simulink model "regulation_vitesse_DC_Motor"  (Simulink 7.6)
settings: Solver=ode23tb  StartTime=0.0  StopTime=0.4  RelTol=1e-3
PreLoadFcn:
  | close all
  | clc
  | clear all
PostLoadFcn:
  | Ki=1e-4;
  | Kd=1e-4;
  | Kp=5;
StopFcn:
  | close all, clc
  | load reg_vit.mat
  | plot(x(1,:),x(2,:), x(1,:),x(3,:))
  | grid
  | title('Consigne et sortie vitesse DC Motor')
  | xlabel('temps')
  | axis([0 0.4 0 1200])
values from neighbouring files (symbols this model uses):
  f = 1e-8    (= 1e-08)    [parametres.m]    (also in impedance_quartz.m = [1.59:0.0005:1.596]*1e6)
  R = 4    [parametres.m]    (also in Prog_callbacks.m = 1000; oscillateur_dephasage.m = 1000; Calcul_Ampl_phase_A.m = 1; circuit_RLC_parallele_.m)
undefined symbols (not defined in the file or in its folder): sigbuilder_block
libraries: fl_lib x19, nesl_utility x6

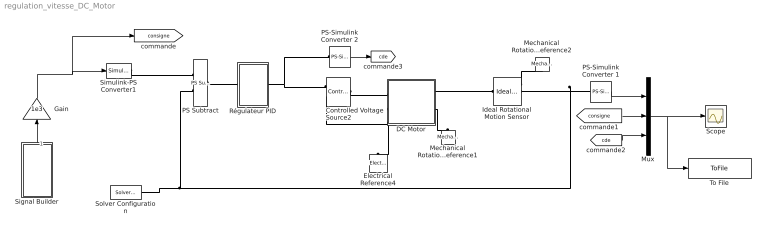
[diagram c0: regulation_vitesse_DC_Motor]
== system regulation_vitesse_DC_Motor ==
  Controlled Voltage Source2 : fl_lib/Electrical/Electrical Sources/Controlled Voltage Source  DialogController=NetworkEngine.DynNeDlgSource  SystemSampleTime=-1  i_Log=off  v_Log=off  LocalVarNames=|current|voltage|power  LocalVarDescs=|Current (A)|Voltage (V)|Power (W)  LocalVarLogging=[0 0 0]
  DC Motor : Subsystem  LoadFcn=|
      | R=4; % Résistance d'induit             
      | L=1e-5; % Inductance d'induit          
      | K=0.0005; % paramètre électromagnétique
      |                                        
      | J=1; %inertie (g*cm^2)                 
      | Cr=0.02e-3; % frottements              
      | f=1e-8; % amortissement
  Electrical Reference4 : fl_lib/Electrical/Electrical Elements/Electrical Reference  DialogController=NetworkEngine.DynNeDlgSource  SystemSampleTime=-1  i_Log=off  LocalVarNames=|i  LocalVarDescs=|i  LocalVarLogging=[]
  Gain : Gain  Gain=1e3
  Ideal Rotational Motion Sensor : fl_lib/Mechanical/Mechanical Sensors/Ideal Rotational Motion Sensor  DialogController=NetworkEngine.DynNeDlgSource  SystemSampleTime=-1  offset=0 rad  w_Log=off  t_Log=off  phi_Log=off  LocalVarNames=|w|t|phi  LocalVarDescs=|w|t|phi  LocalVarLogging=[0 0 0]
  Mechanical Rotational Reference1 : fl_lib/Mechanical/Rotational Elements/Mechanical Rotational Reference  DialogController=NetworkEngine.DynNeDlgSource  SystemSampleTime=-1  t_Log=off  LocalVarNames=|t  LocalVarDescs=|t  LocalVarLogging=[]
  Mechanical Rotational Reference2 : fl_lib/Mechanical/Rotational Elements/Mechanical Rotational Reference  DialogController=NetworkEngine.DynNeDlgSource  SystemSampleTime=-1  t_Log=off  LocalVarNames=|t  LocalVarDescs=|t  LocalVarLogging=[]
  Mux : Mux  Inputs=3
  PS Subtract : fl_lib/Physical Signals/Functions/PS Subtract  DialogController=NetworkEngine.DynNeDlgSource  SystemSampleTime=-1  LocalVarLogging=[]
  PS-Simulink Converter 1 : nesl_utility/PS-Simulink Converter  DialogController=NetworkEngine.DynNeUtilDlgSource  SystemSampleTime=-1  PhysicalDomain=network_engine_domain  LeftPortType=input  RightPortType=output  SubClassName=ps_output  Unit=1  AffineConversion=off
  PS-Simulink Converter 2 : nesl_utility/PS-Simulink Converter  DialogController=NetworkEngine.DynNeUtilDlgSource  SystemSampleTime=-1  PhysicalDomain=network_engine_domain  LeftPortType=input  RightPortType=output  SubClassName=ps_output  Unit=1  AffineConversion=off
  Régulateur PID : Subsystem
  Scope : Scope
  Signal Builder : Subsystem  Tag=STV Subsys  LoadFcn=sigbuilder_block('load');  StartFcn=sigbuilder_block('start');  StopFcn=sigbuilder_block('stop');  ClipboardFcn=sigbuilder_block('clipboard');
  Simulink-PS Converter1 : nesl_utility/Simulink-PS Converter  DialogController=NetworkEngine.DynNeUtilDlgSource  SystemSampleTime=-1  PhysicalDomain=network_engine_domain  LeftPortType=input  RightPortType=output  SubClassName=ps_input  Unit=1  AffineConversion=off  InputFilterTimeConstant=.001  UdotUserProvided=0
  Solver Configuration : nesl_utility/Solver Configuration  DialogController=NetworkEngine.DynNeUtilDlgSource  SystemSampleTime=-1  PhysicalDomain=network_engine_domain  LeftPortType=input  RightPortType=generic  SubClassName=solver  Accelerate=off  Profile=off  ResidualTolerance=1e-9  MaxNonlinIter=12  MaxModeIter=2  DoFixedCost=off  UseLocalSampling=off  DoDC=off  LinearAlgebra=Full  LocalSolverSampleTime=.001  LocalSolverChoice=NE_BACKWARD_EULER_ADVANCER  UseLocalSolver=off
  To File : ToFile  Filename=reg_vit.mat  MatrixName=x
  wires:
  PS-Simulink Converter 1/1 -> Mux/1
  Mux/1 -> To File/1, Scope/1
  Gain/1 -> Simulink-PS Converter1/1, [consigne]
  [consigne] -> Mux/2
  PS-Simulink Converter 2/1 -> [cde]
  [cde] -> Mux/3
  Signal Builder/1(Signal 2) -> Gain/1
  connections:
  Ideal Rotational Motion Sensor/RConn1 -- Mechanical Rotational Reference2/LConn1
  PS Subtract/LConn2 -- PS-Simulink Converter 1/LConn1 -- Ideal Rotational Motion Sensor/RConn2 -- Solver Configuration/RConn1
  DC Motor/RConn1 -- Ideal Rotational Motion Sensor/LConn1
  DC Motor/LConn2 -- Electrical Reference4/LConn1 -- Controlled Voltage Source2/RConn2
  Régulateur PID/RConn1 -- Controlled Voltage Source2/RConn1 -- PS-Simulink Converter 2/LConn1
  Controlled Voltage Source2/LConn1 -- DC Motor/LConn1
  Simulink-PS Converter1/RConn1 -- PS Subtract/LConn1
  PS Subtract/RConn1 -- Régulateur PID/LConn1
  DC Motor/RConn2 -- Mechanical Rotational Reference1/LConn1

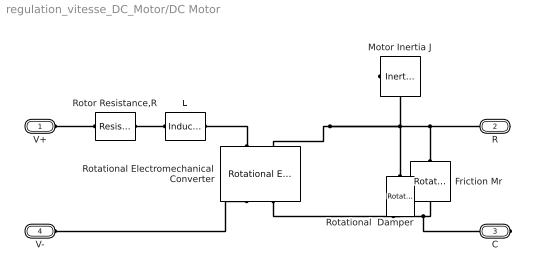
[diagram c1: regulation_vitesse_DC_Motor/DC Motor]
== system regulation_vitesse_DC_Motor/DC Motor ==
  Friction Mr : fl_lib/Mechanical/Rotational Elements/Rotational Friction  DialogController=NetworkEngine.DynNeDlgSource  SystemSampleTime=-1  brkwy_trq=Cr N*m  Col_trq=Cr N*m  visc_coef=0 N*m/(rad/s)  trans_coef=10 s/rad  vel_thr=0.1 rad/s  t_Log=off  w_Log=off  LocalVarNames=|friction_torque|rel_velocity|power  LocalVarDescs=|Friction torque (N*m)|Relative velocity (rad/s)|Power (W)  LocalVarLogging=[0 0 0]
  L : fl_lib/Electrical/Electrical Elements/Inductor  DialogController=NetworkEngine.DynNeDlgSource  SystemSampleTime=-1  l=L H  i0=0 A  r=0 Ohm  g=1e-09 1/Ohm  i_Log=off  v_Log=off  i_L_Log=off  LocalVarNames=|current|voltage|power  LocalVarDescs=|Inductor current (A) |Voltage across inductor (V)|Power (W)  LocalVarLogging=[0 0 0]
  Motor Inertia J : fl_lib/Mechanical/Rotational Elements/Inertia  DialogController=NetworkEngine.DynNeDlgSource  SystemSampleTime=-1  inertia=J g*cm^2  initial_velocity=0 rad/s  t_Log=off  LocalVarNames=|torque|velocity  LocalVarDescs=|Inertia torque (N*m)|Inertia absolute velocity (rad/s)  LocalVarLogging=[0 0]
  Rotational Electromechanical Converter : fl_lib/Electrical/Electrical Elements/Rotational Electromechanical Converter  DialogController=NetworkEngine.DynNeDlgSource  SystemSampleTime=-1  K=1e-5 V/(rad/s)  i_Log=off  v_Log=off  t_Log=off  w_Log=off  LocalVarNames=|current|voltage|power|torque|speed  LocalVarDescs=|Current (A)|Voltage (V)|Power (W)|Torque (Nm)|Angular speed (rad/s)  LocalVarLogging=[0 0 0 0 0]
  Rotational  Damper : fl_lib/Mechanical/Rotational Elements/Rotational Damper  DialogController=NetworkEngine.DynNeDlgSource  SystemSampleTime=-1  D=f N*m/(rad/s)  t_Log=off  w_Log=off  LocalVarNames=|t|w  LocalVarDescs=|t|w  LocalVarLogging=[0 0]
  Rotor Resistance,R : fl_lib/Electrical/Electrical Elements/Resistor  Tag=Factory Generic  DialogController=NetworkEngine.DynNeDlgSource  SystemSampleTime=-1  R=R Ohm  i_Log=off  v_Log=off  LocalVarNames=|current|voltage|power  LocalVarDescs=|Resistor current (A)|Voltage across resistor (V)|Power (W)  LocalVarLogging=[0 0 0]
  V+ : PMIOPort  Port=1  Side=Left
  R : PMIOPort  Port=2  Side=Right
  C : PMIOPort  Port=3  Side=Right
  V- : PMIOPort  Port=4  Side=Left
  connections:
  Rotational Electromechanical Converter/RConn2 -- Friction Mr/RConn1 -- C/RConn1 -- Rotational  Damper/RConn1
  Motor Inertia J/LConn1 -- Rotational Electromechanical Converter/LConn2 -- Friction Mr/LConn1 -- R/RConn1 -- Rotational  Damper/LConn1
  L/LConn1 -- Rotor Resistance,R/RConn1
  Rotor Resistance,R/LConn1 -- V+/RConn1
  V-/RConn1 -- Rotational Electromechanical Converter/RConn1
  Rotational Electromechanical Converter/LConn1 -- L/RConn1

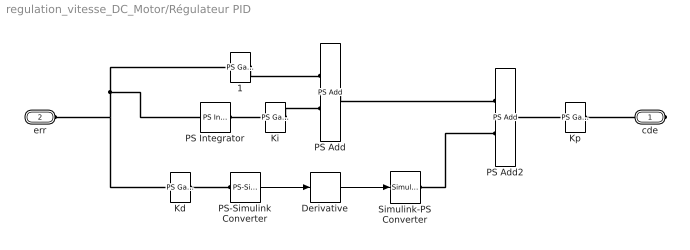
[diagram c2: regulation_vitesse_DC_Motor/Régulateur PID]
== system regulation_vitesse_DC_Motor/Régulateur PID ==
  1 : fl_lib/Physical Signals/Functions/PS Gain  DialogController=NetworkEngine.DynNeDlgSource  SystemSampleTime=-1  gain=1  LocalVarLogging=[]
  Derivative : Derivative
  Kd : fl_lib/Physical Signals/Functions/PS Gain  DialogController=NetworkEngine.DynNeDlgSource  SystemSampleTime=-1  gain=Kd  LocalVarLogging=[]
  Ki : fl_lib/Physical Signals/Functions/PS Gain  DialogController=NetworkEngine.DynNeDlgSource  SystemSampleTime=-1  gain=Ki  LocalVarLogging=[]
  Kp : fl_lib/Physical Signals/Functions/PS Gain  DialogController=NetworkEngine.DynNeDlgSource  SystemSampleTime=-1  gain=Kp  LocalVarLogging=[]
  PS Add : fl_lib/Physical Signals/Functions/PS Add  DialogController=NetworkEngine.DynNeDlgSource  SystemSampleTime=-1  LocalVarLogging=[]
  PS Add2 : fl_lib/Physical Signals/Functions/PS Add  DialogController=NetworkEngine.DynNeDlgSource  SystemSampleTime=-1  LocalVarLogging=[]
  PS Integrator : fl_lib/Physical Signals/Linear Operators/PS Integrator  DialogController=NetworkEngine.DynNeDlgSource  SystemSampleTime=-1  x0=0  x_Log=off  LocalVarNames=|x  LocalVarDescs=|x  LocalVarLogging=0
  PS-Simulink Converter : nesl_utility/PS-Simulink Converter  DialogController=NetworkEngine.DynNeUtilDlgSource  SystemSampleTime=-1  PhysicalDomain=network_engine_domain  LeftPortType=input  RightPortType=output  SubClassName=ps_output  Unit=1  AffineConversion=off
  Simulink-PS Converter : nesl_utility/Simulink-PS Converter  DialogController=NetworkEngine.DynNeUtilDlgSource  SystemSampleTime=-1  PhysicalDomain=network_engine_domain  LeftPortType=input  RightPortType=output  SubClassName=ps_input  Unit=1  AffineConversion=off  InputFilterTimeConstant=.001  UdotUserProvided=0
  cde : PMIOPort  Port=1  Side=Right
  err : PMIOPort  Port=2  Side=Left
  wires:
  PS-Simulink Converter/1 -> Derivative/1
  Derivative/1 -> Simulink-PS Converter/1
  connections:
  Simulink-PS Converter/RConn1 -- PS Add2/LConn2
  PS Add/RConn1 -- PS Add2/LConn1
  1/RConn1 -- PS Add/LConn1
  Ki/RConn1 -- PS Add/LConn2
  PS Integrator/RConn1 -- Ki/LConn1
  err/RConn1 -- 1/LConn1 -- PS Integrator/LConn1 -- Kd/LConn1
  Kd/RConn1 -- PS-Simulink Converter/LConn1
  Kp/RConn1 -- cde/RConn1
  PS Add2/RConn1 -- Kp/LConn1

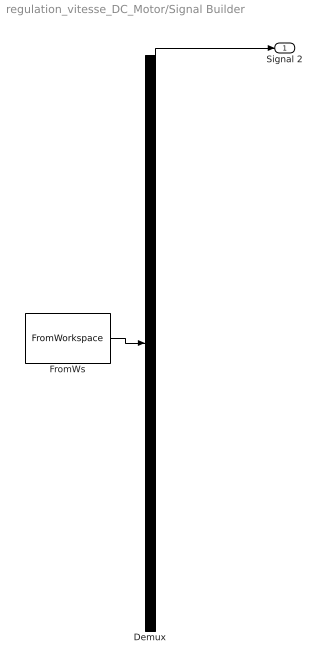
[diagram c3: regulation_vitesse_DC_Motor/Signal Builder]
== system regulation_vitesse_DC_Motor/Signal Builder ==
  Demux : Demux  Tag=STV Demux  Outputs=1
  FromWs : FromWorkspace  Tag=STV FromWs  VariableName=tuvar  SampleTime=0  SigBuilderData=DataTag0  VnvData=DataTag1
  Signal 2 : Outport  Tag=STV Outport
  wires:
  Demux/1 -> Signal 2/1
  FromWs/1 -> Demux/1
